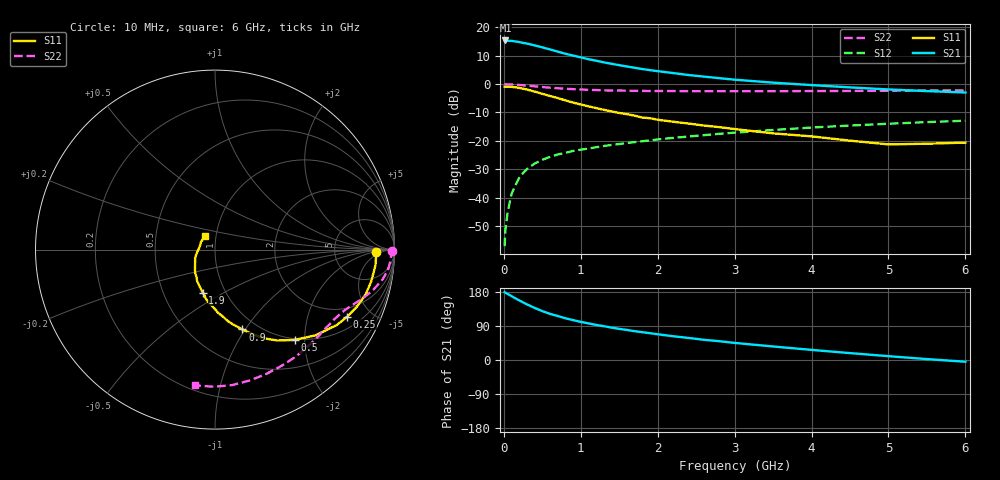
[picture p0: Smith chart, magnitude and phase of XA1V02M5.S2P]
! SIEMENS Discrete & RF Semiconductors
! BFY180
! Si NPN RF Bipolar Junction Transistor in MICRO-X
! VCE = 1 V  IC = 2.5 mA
! Common Emitter S-Parameters:  May  1997
# GHz  S  MA  R  50
!  f  S11  S21  S12  S22
! GHz  MAG  ANG  MAG  ANG  MAG  ANG  MAG  ANG
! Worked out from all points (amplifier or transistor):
!   36 points, 10 MHz to 6 GHz, reference 50 ohm
!   highest |S21| = 15.3 dB at 20 MHz (marker M1)
!   |S21| within 3 dB of that: start of sweep to 577.4 MHz
!   unconditionally stable (mu >= 1): 1.142 GHz to end of sweep
!   at 250 MHz: K = 0.29, MSG = 22.9 dB, |S12| = -31.3 dB
!   at 1.4 GHz: K = 1.11, MAG = 12.2 dB, |S12| = -21.5 dB
!   at 6 GHz: K = 1.30, MAG = 1.7 dB, |S12| = -12.9 dB
!   S11 on the Smith chart (normalised r, x): 10 MHz: 18, -3; 250 MHz: 1.52, -3.58; 500 MHz: 0.98, -1.79; 900 MHz: 0.85, -0.97; 1.9 GHz: 0.78, -0.40; 6 GHz: 0.88, +0.13
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0.01  0.8973 -1.0  5.734 179.0  0.0014 88.8  0.9834 -0.3
0.02  0.8981 -2.3  5.829 177.5  0.0027 91.8  0.9935 -0.9
0.05  0.8982 -5.6  5.741 174.3  0.0056 83.9  0.9819 -2.1
0.1  0.8884 -11.5  5.723 168.5  0.0116 84.4  0.9773 -4.3
0.2  0.8518 -22.0  5.465 157.2  0.0222 76.2  0.9602 -8.2
0.25  0.8261 -26.9  5.283 152.1  0.0271 73.3  0.9494 -10.0
0.3  0.7986 -31.7  5.146 146.9  0.0317 70.6  0.9349 -11.5
0.4  0.7357 -40.5  4.77 137.4  0.0398 65.9  0.9091 -14.3
0.5  0.6707 -48.6  4.412 129.1  0.0463 61.7  0.8826 -16.8
0.6  0.6154 -55.4  4.047 121.8  0.0521 58.9  0.8601 -18.7
0.7  0.5656 -61.0  3.713 116.2  0.0575 56.6  0.8413 -20.5
0.8  0.5146 -66.2  3.4 110.1  0.0614 54.8  0.8235 -22.1
0.9  0.47 -71.1  3.161 105.3  0.0662 53.3  0.8104 -23.5
1.1  0.404 -79.9  2.729 96.6  0.0731 51.0  0.7885 -26.4
1.5  0.3089 -94.0  2.144 82.1  0.0878 48.3  0.7644 -32.0
1.9  0.2497 -106.0  1.751 70.7  0.1015 46.1  0.7527 -37.7
2.2  0.2167 -114.4  1.557 62.7  0.1126 44.4  0.7499 -42.3
3  0.1609 -133.9  1.19 45.1  0.1393 39.2  0.7465 -53.8
3.5  0.1352 -145.2  1.055 35.7  0.1551 35.9  0.7465 -60.9
4.5  0.1007 -171.5  0.871 18.2  0.1857 28.0  0.7545 -75.4
5.5  0.0889 152.5  0.749 2.4  0.2133 19.6  0.764 -90.6
6  0.093 127.7  0.708 -4.6  0.2257 15.1  0.7642 -98.2
